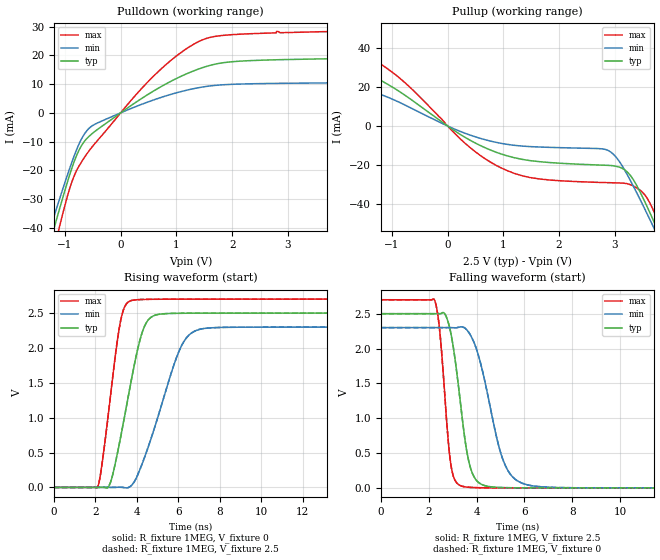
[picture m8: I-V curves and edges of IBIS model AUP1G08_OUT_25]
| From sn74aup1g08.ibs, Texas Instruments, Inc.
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[Model]   AUP1G08_OUT_25
Model_type  Output
Vref =   0
Rref =   1E6
Cref =   30p
Vmeas =   1.25
| variable   typ   min   max
C_comp   2.91pF   2.03pF   4.21pF
| C_pullup   3.24pF   2.03pF   4.21pF
| C_pulldown   2.58pF   2.28pF   3.16pF
[Temperature Range]   40   100   -40
| Ambient temperature   25   85   -40
[Voltage range]   2.5   2.3   2.7
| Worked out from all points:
|   slope of the pulldown table from 0 to 0.375 V, typ, clamps not added: 75.2 ohm
|   slope of the pullup table from 0 to 0.375 V, typ, clamps not added: 55.1 ohm
|   rising waveform, R_fixture 1MEG, V_fixture 0: 20-80 % time 983ps typ, 1.48ns min, 673ps max; typ from 0 V to 2.5 V
|   falling waveform, R_fixture 1MEG, V_fixture 2.5: 20-80 % time 568ps typ, 919ps min, 366ps max; typ from 2.5 V to 0 V
|   rising waveform, R_fixture 1MEG, V_fixture 2.5: 20-80 % time 983ps typ, 1.48ns min, 673ps max; typ from 0 V to 2.5 V
|   falling waveform, R_fixture 1MEG, V_fixture 0: 20-80 % time 568ps typ, 919ps min, 366ps max; typ from 2.5 V to 0 V
[Pulldown]
| AUP1G08_OUT_25
|   Voltage   I(typ)   I(min)   I(max)
-3.6V     -214.2mA   -193.6mA   -239.8mA
-1.26V    -44.57mA   -39.94mA   -52.43mA
-1.205V   -40.76mA   -36.54mA   -48.03mA
-1.115V   -34.59mA   -31.04mA   -40.92mA
-800mV    -15.22mA   -13.23mA   -20.4mA
-685mV    -10.84mA   -8.45mA    -16.54mA
-540mV    -7.689mA   -4.912mA   -12.5mA
675mV     8.558mA    5.038mA    14.35mA
1.105V    12.9mA     7.5mA      21.28mA
1.52V     16.03mA    9.129mA    25.76mA
2.805V    18.45mA    10.24mA    28.28mA
7.2V      19.61mA    10.73mA    29.61mA
[Pullup]
| AUP1G08_OUT_25
|   Voltage   I(typ)   I(min)   I(max)
-3.6V     37.27mA    23.46mA    50.39mA
-2.36V    24.67mA    15.19mA    35.64mA
-1.425V   26mA       17.18mA    35.59mA
-760mV    15.58mA    10.62mA    21.96mA
405mV     -7.279mA   -4.651mA   -11.04mA
1.05V     -15.07mA   -9.293mA   -22.54mA
2.845V    -20.04mA   -12.07mA   -28.88mA
3.17V     -22.17mA   -22.1mA    -29.2mA
3.455V    -33.68mA   -37.5mA    -32.73mA
3.685V    -47.63mA   -50.96mA   -42.51mA
3.82V     -56.3mA    -59.07mA   -51.48mA
7.2V      -294.9mA   -278.9mA   -311.6mA
[Ramp]
| AUP1G08_OUT_25
| variable   typ   min   max
dV/dt_r   1.50/9.88E-10   1.38/1.48E-09   1.62/6.75E-10
dV/dt_f   1.51/5.76E-10   1.39/9.25E-10   1.63/3.70E-10
R_load = 1MEG
[Rising Waveform]
| AUP1G08_OUT_25
R_fixture =   1MEG
C_fixture =   0
L_fixture =   0
V_fixture =   0
V_fixture_min = 0
V_fixture_max = 0
|   Time   V(typ)   V(min)   V(max)
0s        23.72nV    103.4nV    1.644nV
2.125ns   -48.33uV   1.454uV    16.88mV
2.685ns   37.6mV     -92.03uV   1.194V
3.18ns    659.9mV    1.885mV    2.327V
3.74ns    1.545V     27.48mV    2.68V
4.205ns   2.171V     297.8mV    2.695V
4.6ns     2.418V     623.8mV    2.697V
6.05ns    2.497V     1.964V     2.699V
6.985ns   2.498V     2.263V     2.7V
29.99ns   2.5V       2.3V       2.7V
[Falling Waveform]
| AUP1G08_OUT_25
R_fixture =   1MEG
C_fixture =   0
L_fixture =   0
V_fixture =   2.5
V_fixture_min = 2.3
V_fixture_max = 2.7
|   Time   V(typ)   V(min)   V(max)
0s        2.5V       2.3V       2.7V
2.255ns   2.5V       2.3V       2.69V
2.47ns    2.5V       2.3V       2.234V
2.93ns    2.218V     2.3V       336.1mV
3.43ns    927.2mV    2.308V     20.79mV
3.705ns   342.3mV    2.217V     7.734mV
4.04ns    91.56mV    1.947V     2.675mV
5.115ns   3.73mV     394.7mV    234uV
6.11ns    528.6uV    44.64mV    128.3uV
29.99ns   179uV      276.3uV    112.6uV
[Rising Waveform]
| AUP1G08_OUT_25
R_fixture =   1MEG
C_fixture =   0
L_fixture =   0
V_fixture =   2.5
V_fixture_min = 2.3
V_fixture_max = 2.7
|   Time   V(typ)   V(min)   V(max)
0s        178.6uV    276.1uV    112.4uV
2.125ns   130.2uV    277.4uV    17mV
2.685ns   37.82mV    184uV      1.195V
3.18ns    660.6mV    2.161mV    2.328V
3.74ns    1.546V     27.82mV    2.68V
4.205ns   2.172V     298.5mV    2.695V
4.6ns     2.418V     624.9mV    2.697V
6.05ns    2.497V     1.965V     2.699V
6.98ns    2.498V     2.263V     2.7V
29.99ns   2.5V       2.3V       2.7V
[Falling Waveform]
| AUP1G08_OUT_25
R_fixture =   1MEG
C_fixture =   0
L_fixture =   0
V_fixture =   0
V_fixture_min = 0
V_fixture_max = 0
|   Time   V(typ)   V(min)   V(max)
0s        2.5V       2.3V       2.7V
2.255ns   2.5V       2.3V       2.69V
2.47ns    2.5V       2.3V       2.233V
2.93ns    2.218V     2.3V       335.8mV
3.43ns    926.6mV    2.308V     20.66mV
3.705ns   341.8mV    2.217V     7.615mV
4.04ns    91.28mV    1.947V     2.56mV
5.115ns   3.542mV    393.9mV    121.2uV
6.11ns    348.1uV    44.18mV    15.9uV
29.99ns   424.2nV    293.1nV    222.2nV
